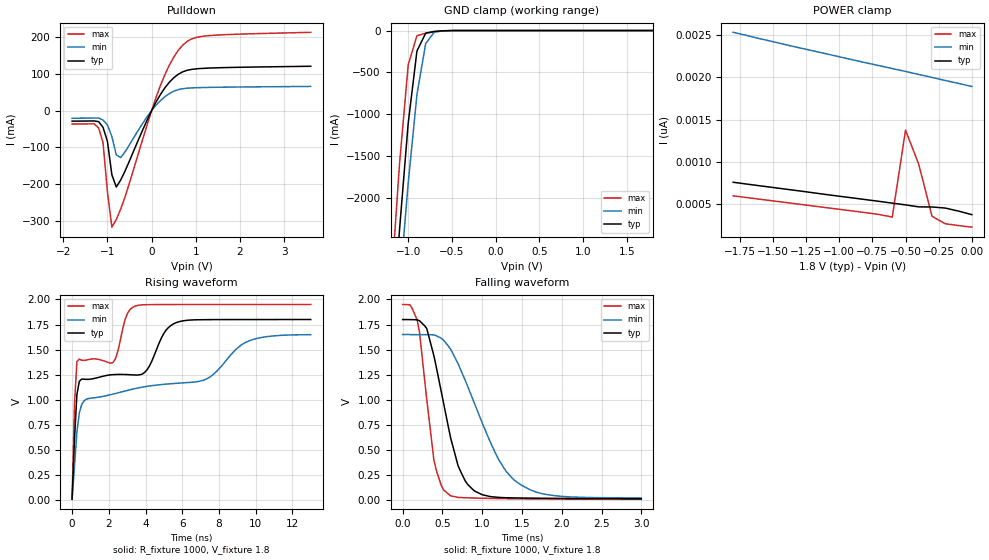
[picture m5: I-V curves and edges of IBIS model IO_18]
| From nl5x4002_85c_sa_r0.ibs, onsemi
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[Model]   IO_18
Model_type I/O_open_drain
Enable Active-High
Polarity Non-Inverting
Vinh=1.26
Vinl=0.54
Vref=1.8
Vmeas=0.9
Rref=1000
Cref=50p
C_comp   6.0p   NA   NA
[Model Spec]
Vinh   1.26   1.155   1.365
Vinl   0.54   0.495   0.585
Vmeas   0.9   0.825   0.975
[Temperature Range] 25   85   -40
[Voltage Range]   1.8   1.65   1.95
[POWER Clamp Reference]  1.8   1.65   1.95
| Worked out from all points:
|   slope of the pulldown table from 0 to 0.27 V, typ, clamps not added: 4.78 ohm
|   GND clamp passes 1 mA (typ) near -0.51 V on its own axis
|   falling waveform, R_fixture 1000, V_fixture 1.8: 20-80 % time 296ps typ, 536ps min, 166ps max; typ from 1.8 V to 0.01 V
|   rising waveform, R_fixture 1000, V_fixture 1.8: 20-80 % time 4.39ns typ, 7.94ns min, 2.54ns max; typ from 0.007 V to 1.8 V
[Pulldown]
-1.8V     -28.8mA    -20.94mA   -36.59mA
-1.2V     -30.11mA   -20.16mA   -47.29mA
-1.1V     -45.62mA   -25.7mA    -86.92mA
-1V       -83.93mA   -39.29mA   -221.5mA
-900mV    -174.8mA   -70.48mA   -317.5mA
-800mV    -208.1mA   -120.6mA   -296.8mA
-700mV    -189.1mA   -128.1mA   -268mA
200mV     43.97mA    27.35mA    68.63mA
500mV     89.22mA    52.62mA    145.4mA
700mV     105.3mA    59.53mA    177.8mA
1.2V      115.2mA    62.83mA    202.9mA
3.6V      120.7mA    65.78mA    213.1mA
[GND Clamp]
-1.8V     -12.82A    -12.63A    -13.11A
-1.2V     -3.822A    -4.412A    -3.136A
-1.1V     -2.385A    -3.071A    -1.6A
-1V       -1.105A    -1.818A    -410.1mA
-900mV    -244.1mA   -763.4mA   -62.39mA
-800mV    -31.41mA   -154.3mA   -31.83mA
-700mV    -10.05mA   -17.99mA   -15.56mA
-500mV    -634.4uA   -553uA     -616uA
1.8V      369.7pA    1.892nA    221pA
[POWER Clamp]
-1.8V     754.6pA    2.536nA    593.1pA
-1.4V     671.8pA    2.388nA    513.3pA
-800mV    548.1pA    2.175nA    393.2pA
-700mV    527.7pA    2.14nA     371.5pA
-600mV    506.5pA    2.106nA    341.2pA
-500mV    485.8pA    2.071nA    1.374nA
-400mV    462pA      2.036nA    967.1pA
-300mV    460.8pA    2nA        350.2pA
-200mV    447.8pA    1.964nA    261pA
0V        369.8pA    1.892nA    221pA
[Falling Waveform]
R_fixture=1000
V_fixture=1.8
V_fixture_min=1.65
V_fixture_max=1.95
0s        1.8V       1.65V      1.95V
181.8ps   1.797V     1.649V     1.798V
303ps     1.711V     1.649V     1.004V
393.9ps   1.435V     1.647V     392.3mV
575.8ps   724.4mV    1.534V     57.7mV
818.2ps   153.5mV    1.132V     20.07mV
1.182ns   26.16mV    441.6mV    13.42mV
1.394ns   19.52mV    203.3mV    10.97mV
1.879ns   15.1mV     45.13mV    8.678mV
3ns       10.41mV    18.92mV    5.282mV
[Rising Waveform]
R_fixture=1000
V_fixture=1.8
V_fixture_min=1.65
V_fixture_max=1.95
0s        7.29mV     10.46mV    5.18mV
131.3ps   604.6mV    331.5mV    957.3mV
262.6ps   1.05V      678.9mV    1.38V
656.6ps   1.205V     989.3mV    1.392V
2.232ns   1.25V      1.056V     1.371V
3.283ns   1.248V     1.104V     1.92V
5.778ns   1.776V     1.165V     1.95V
7.485ns   1.799V     1.223V     1.95V
9.717ns   1.8V       1.593V     1.95V
13ns      1.8V       1.649V     1.95V
[Ramp]
R_load=1000
dV/dt_r   1.075E+0/1.807E-10   9.830E-1/2.761E-10   1.167E+0/1.224E-10
dV/dt_f   1.071E+0/2.952E-10   9.693E-1/5.274E-10   1.165E+0/1.659E-10
|[End   IO_18
